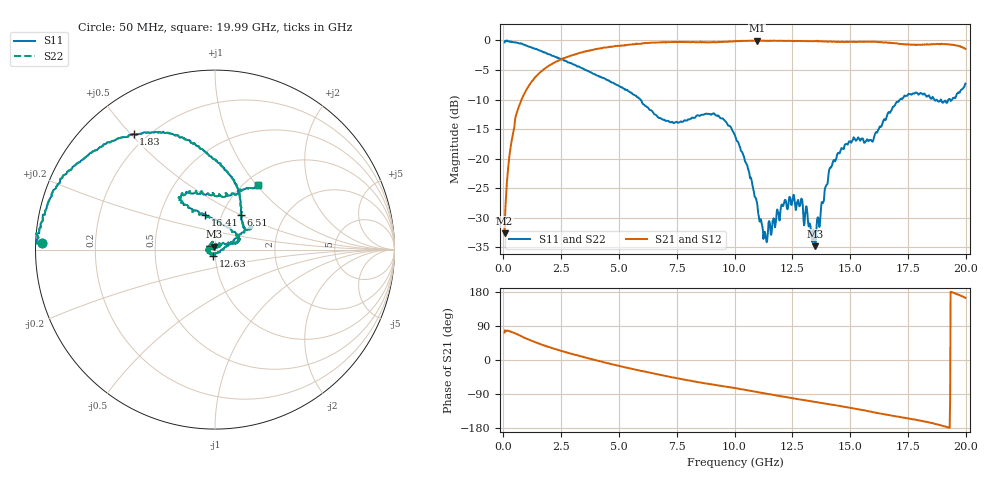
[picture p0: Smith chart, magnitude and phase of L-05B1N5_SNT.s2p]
! Data Taken on a HP 8720C VNA using a shunt-through fixture with TRL* de-embedding
#	mhz	s	ma	r	50
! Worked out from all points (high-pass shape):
!   998 points, 50 MHz to 19.99 GHz, reference 50 ohm
!   highest |S21| = -0.01 dB at 10.97 GHz (marker M1); lowest = -32.6 dB at 50 MHz (marker M2)
!   |S21| within 3 dB of the highest: 2.598 GHz to end of sweep
!   lowest |S11| = -34.8 dB at 13.49 GHz (marker M3), VSWR 1.04, Z = 49.4 + j1.69 ohm
!   |S11| at or under -10 dB: 5.925 GHz to 17.15 GHz (11.22 GHz wide, 97.3 % of centre); 18.65 GHz to 18.93 GHz (282 MHz wide, 1.5 % of centre); 18.93 GHz to 19.25 GHz (318.1 MHz wide, 1.67 % of centre)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
!   |S22| runs from -34.8 to 0.0 dB; largest |S21 - S12| = 0
!   S11 on the Smith chart (normalised r, x): 50 MHz: 0.02, +0.02; 1.83 GHz: 0.15, +0.51; 6.51 GHz: 1.22, +0.50; 12.63 GHz: 0.98, -0.07; 16.41 GHz: 0.84, +0.34; 19.99 GHz: 1.15, +1.02
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50  0.9635 177.8  0.02336 72.7  0.02336 72.7  0.9635 177.8
250  0.9768 172.7  0.1015 76.0  0.1015 76.0  0.9768 172.7
590  0.9596 160.0  0.2484 68.0  0.2484 68.0  0.9596 160.0
1830  0.7876 125.2  0.5861 37.0  0.5861 37.0  0.7876 125.2
3390  0.5843 99.2  0.7935 9.1  0.7935 9.1  0.5843 99.2
6510  0.2401 53.4  0.9592 -35.7  0.9592 -35.7  0.2401 53.4
6710  0.2215 48.8  0.9618 -38.1  0.9618 -38.1  0.2215 48.8
9110  0.2417 31.8  0.9698 -65.4  0.9698 -65.4  0.2417 31.8
10030  0.1555 31.8  0.9849 -74.1  0.9849 -74.1  0.1555 31.8
10970  0.04271 0.5  0.9985 -84.4  0.9985 -84.4  0.04271 0.5
11330  0.02302 -52.5  0.9929 -88.3  0.9929 -88.3  0.02302 -52.5
12130  0.04131 -156.2  0.9922 -96.8  0.9922 -96.8  0.04131 -156.2
12630  0.03921 -106.2  0.9914 -101.9  0.9914 -101.9  0.03921 -106.2
13350  0.02266 138.2  0.9866 -109.6  0.9866 -109.6  0.02266 138.2
13490  0.01821 110.0  0.9869 -110.7  0.9869 -110.7  0.01821 110.0
14130  0.08321 27.6  0.9768 -117.2  0.9768 -117.2  0.08321 27.6
14510  0.1119 19.5  0.9726 -120.6  0.9726 -120.6  0.1119 19.5
16410  0.2012 105.6  0.9613 -142.3  0.9613 -142.3  0.2012 105.6
16670  0.2484 119.0  0.9577 -145.3  0.9577 -145.3  0.2484 119.0
17890  0.3615 120.9  0.9163 -158.4  0.9163 -158.4  0.3615 120.9
19250  0.3161 78.0  0.9271 -178.0  0.9271 -178.0  0.3161 78.0
19990  0.4314 56.1  0.849 163.8  0.849 163.8  0.4314 56.1
